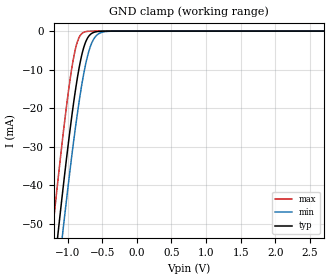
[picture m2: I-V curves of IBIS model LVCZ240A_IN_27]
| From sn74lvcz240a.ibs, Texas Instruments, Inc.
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[Model]   LVCZ240A_IN_27
Model_type  Input
Vinl = 0.8
Vinh = 2
| variable   typ   min   max
C_comp   0.81pF   0.69pF   0.93pF
[Temperature Range]   40   100   -40
| Ambient temperature   25   85   -40
[Voltage range]   2.7   2.7   2.7
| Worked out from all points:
|   GND clamp passes 1 mA (typ) near -0.68 V on its own axis
[GND Clamp]
| LVCZ240A_IN_27
|   Voltage   I(typ)   I(min)   I(max)
-5.5V     -872.3mA   -880mA     -863mA
-1.22V    -65.92mA   -76.78mA   -51.96mA
-1.145V   -53.37mA   -64.25mA   -39.37mA
-1.12V    -49.28mA   -60.14mA   -35.29mA
-1.08V    -42.85mA   -53.67mA   -28.94mA
-1.06V    -39.7mA    -50.49mA   -25.86mA
-960mV    -24.78mA   -35.18mA   -11.94mA
-860mV    -12.16mA   -21.41mA   -2.808mA
-785mV    -5.383mA   -12.75mA   -501uA
-715mV    -1.873mA   -6.62mA    -78.61uA
-570mV    -118uA     -920.2uA   -1.515uA
2.7V      1.113nA    59.61nA    5.15pA
